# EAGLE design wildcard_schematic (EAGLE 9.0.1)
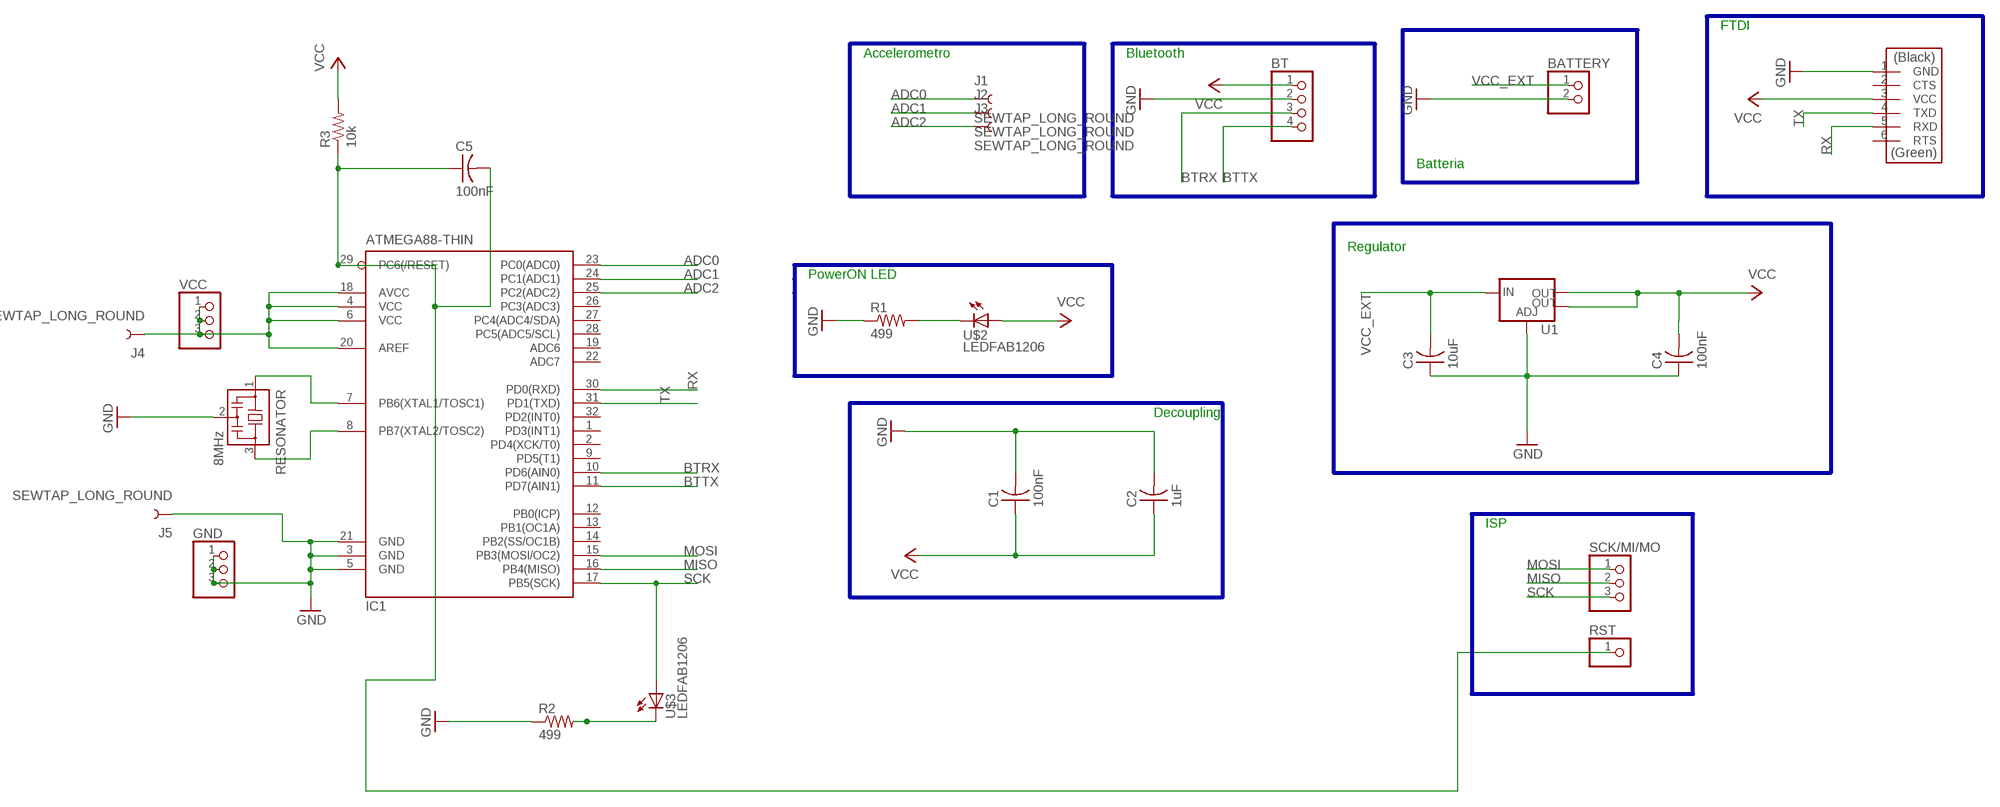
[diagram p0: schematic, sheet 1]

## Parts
BATTERY  PINHD-1X2  [1X02]
BT  PINHD-1X4  [1X04]
C1  100nF  CAP-US1206FAB  [C1206FAB]
C2  1uF  CAP-US1206FAB  [C1206FAB]
C3  10uF  CAP-US1206FAB  [C1206FAB]
C4  100nF  CAP-US1206FAB  [C1206FAB]
C5  100nF  CAP-US1206FAB  [C1206FAB]
GND  PINHD-1X3  [1X03]
IC1  ATMEGA88-THIN  [TQFP32-08THIN]
J1  SEWTAP_LONG_ROUND  [PETAL-LONG-2]
J2  SEWTAP_LONG_ROUND  [PETAL-LONG-2]
J3  SEWTAP_LONG_ROUND  [PETAL-LONG-2]
J4  SEWTAP_LONG_ROUND  [PETAL-LONG-2]
J5  SEWTAP_LONG_ROUND  [PETAL-LONG-2]
R1  499  RES-US1206FAB  [R1206FAB]
R2  499  RES-US1206FAB  [R1206FAB]
R3  10k  RES-US1206FAB  [R1206FAB]
RESONATOR  8MHz  RESONATOR  [EFOBM]
RST  PINHD-1X1  [1X01]
SCK/MI/MO  PINHD-1X3  [1X03]
U1  V_REG_LM1117SOT223  [SOT223]
U$2  LEDFAB1206  [LED1206FAB]
U$3  LEDFAB1206  [LED1206FAB]
U$4  FTDI-SMD-HEADER  [1X06SMD]
VCC  PINHD-1X3  [1X03]

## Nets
ADC0: IC1.23(PC0(ADC0)) J1.1
ADC1: IC1.24(PC1(ADC1)) J2.1
ADC2: IC1.25(PC2(ADC2)) J3.1
BTRX: BT.3 IC1.10(PD6(AIN0))
BTTX: BT.4 IC1.11(PD7(AIN1))
GND: BATTERY.2 BT.2 C1.2 C2.2 C3.1 C4.1 GND.1 GND.2 GND.3 IC1.3(GND) IC1.5(GND) IC1.21(GND) J5.1 R1.1 R2.1 RESONATOR.2 U1.1(ADJ) U$4.1(GND)
MISO: IC1.16(PB4(MISO)) SCK/MI/MO.2
MOSI: IC1.15(PB3(MOSI/OC2)) SCK/MI/MO.1
N$1: IC1.4(VCC) IC1.6(VCC) IC1.18(AVCC) IC1.20(AREF) J4.1 VCC.1 VCC.2 VCC.3
N$2: C5.1 C5.2 IC1.29(PC6(/RESET)) R3.1 RST.1
N$7: IC1.7(PB6(XTAL1/TOSC1)) RESONATOR.1
N$8: IC1.8(PB7(XTAL2/TOSC2)) RESONATOR.3
N$23: R2.2 U$3.2(C)
N$24: R1.2 U$2.2(C)
RX: IC1.30(PD0(RXD)) U$4.5(RXD)
SCK: IC1.17(PB5(SCK)) SCK/MI/MO.3 U$3.1(A)
TX: IC1.31(PD1(TXD)) U$4.4(TXD)
VCC: BT.1 C1.1 C2.1 C4.2 R3.2 U1.2(OUT) U1.4(OUT) U$2.1(A) U$4.3(VCC)
VCC_EXT: BATTERY.1 C3.2 U1.3(IN)
Unconnected: IC1.1(PD3(INT1)) IC1.2(PD4(XCK/T0)) IC1.9(PD5(T1)) IC1.12(PB0(ICP)) IC1.13(PB1(OC1A)) IC1.14(PB2(SS/OC1B)) IC1.19(ADC6) IC1.22(ADC7) IC1.26(PC3(ADC3)) IC1.27(PC4(ADC4/SDA)) IC1.28(PC5(ADC5/SCL)) IC1.32(PD2(INT0)) U$4.2(CTS) U$4.6(RTS)

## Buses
B$1
B$2
B$3
B$4
B$5
B$6
B$7
B$8

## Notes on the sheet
- FTDI
- Accelerometro | Bluetooth
- Batteria
- Regulator
- PowerON LED
- Decoupling
- ISP

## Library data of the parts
BATTERY = pinhead:PINHD-1X2: PIN HEADER
BT = pinhead:PINHD-1X4: PIN HEADER
C1-C5 = fab:CAP-US
GND SCK/MI/MO VCC = pinhead:PINHD-1X3: PIN HEADER
IC1 = fab:ATMEGA88-THIN
J1-J5 = LilyPad-Wearables:SEWTAP: SparkFun LilyPad Sew Taps
R1-R3 = fab:RES-US: Resistor (US Symbol)
RESONATOR = fab:RESONATOR
RST = pinhead:PINHD-1X1: PIN HEADER
U1 = fab:V_REG_LM1117: Voltage Regulator LM1117 Standard adjustable voltage regulator but in SMD form. Spark Fun Electronics SKU : COM-00595; PROD_ID: VREG-08170
U$2 U$3 = fab:LED: LED
U$4 = fab:FTDI-SMD-HEADER

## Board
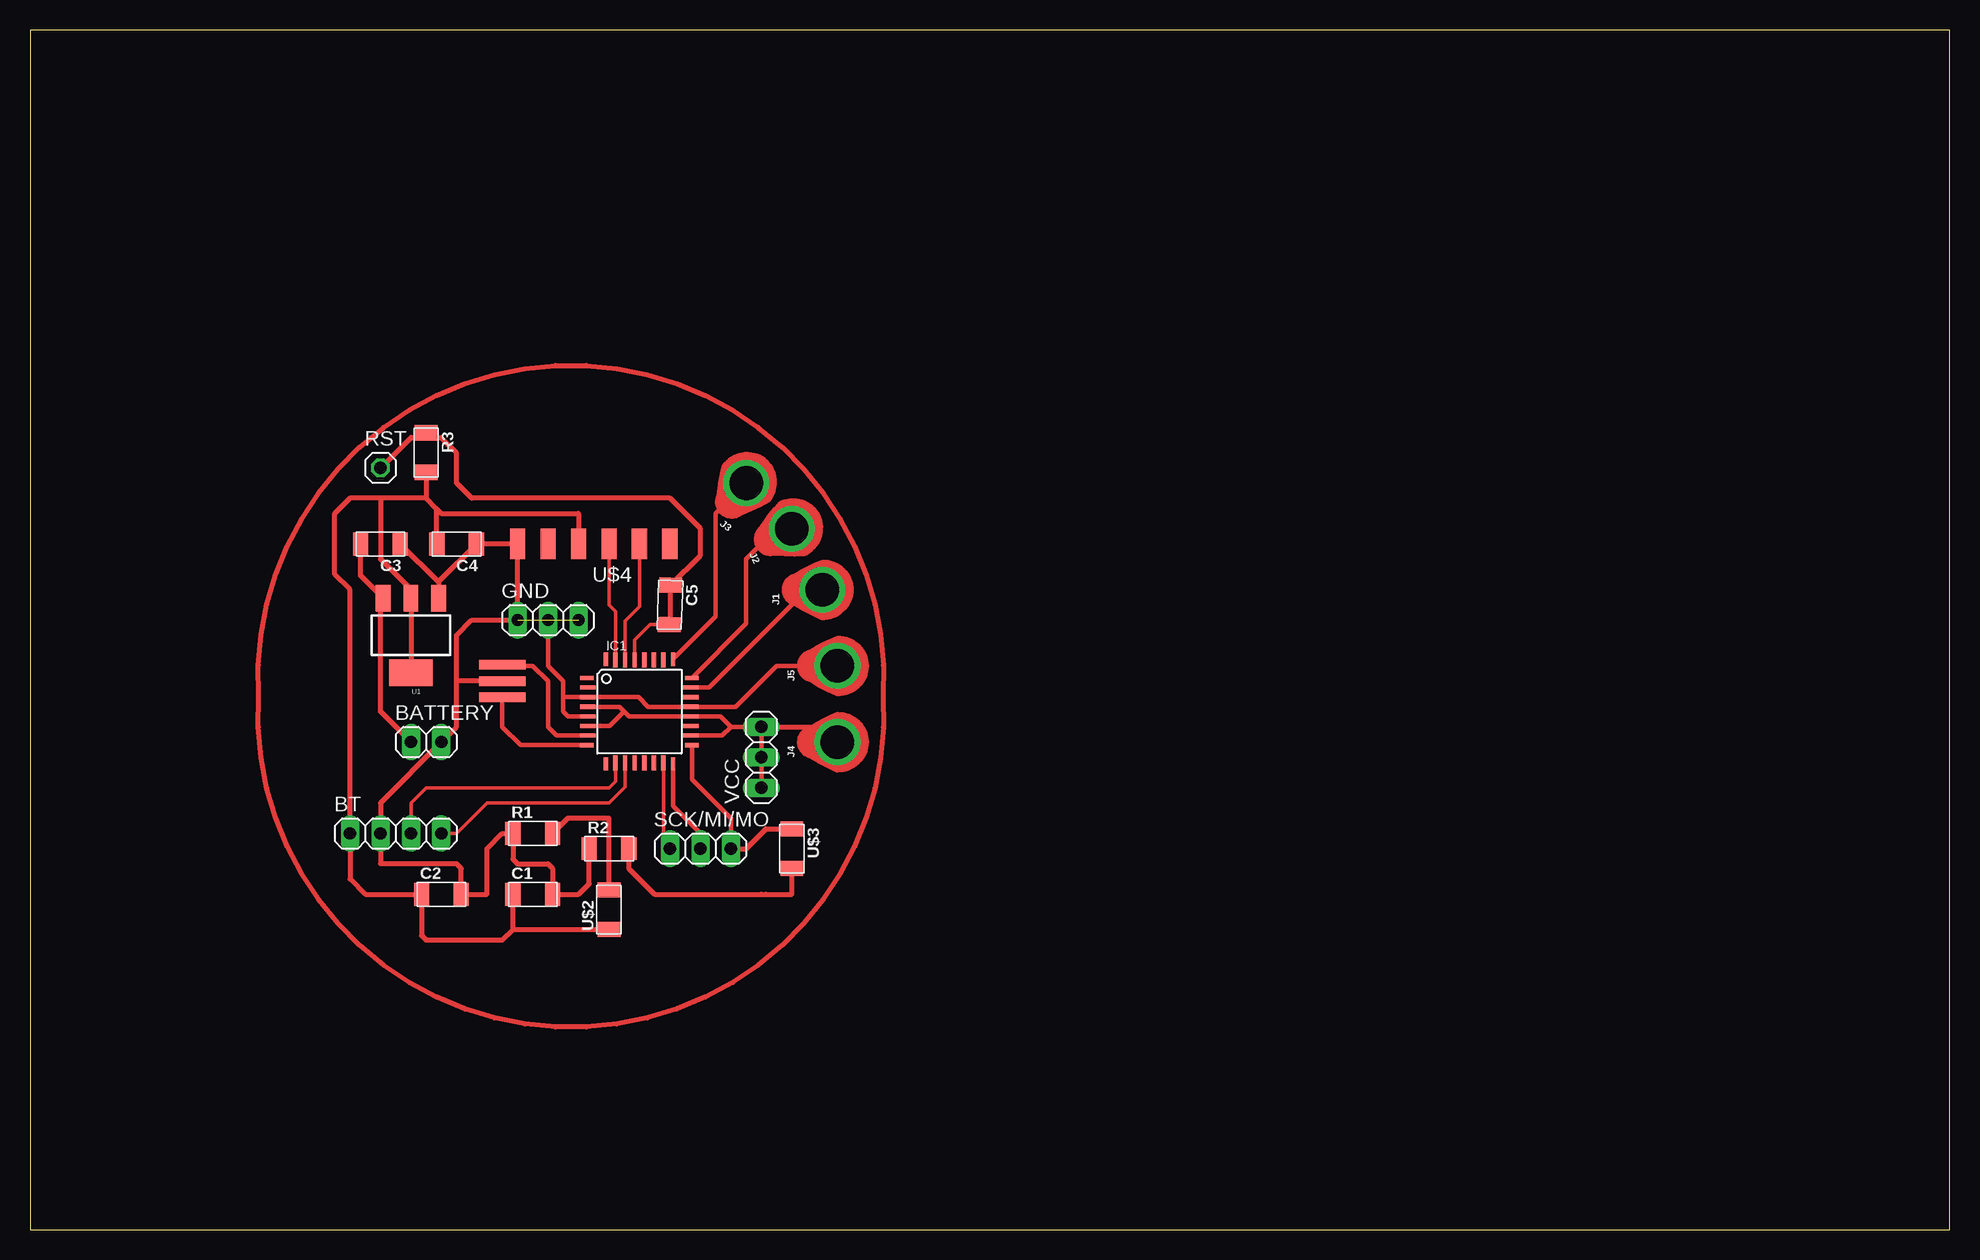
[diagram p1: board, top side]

Size 160 x 100 mm. Coordinates in mm from the lower left corner, seen from the top.
Outline: 0,0 160,0 160,100 0,100 0,0
Copper layers (1*16): Top 0.035mm / dielectric 1.5mm / Bottom 0.035mm
Design rules "default": minimum track width 6mil, minimum drill 0.35mm, track to track 6mil, track to pad 6mil, pad to pad 6mil, via to via 6mil, smd to smd 6mil, copper to edge 40mil, drill to drill 6mil, minimum pad ring 10mil, minimum via ring 8mil, stop-mask expansion 4mil, vias tented up to drill 0mil, thermal gap 10mil

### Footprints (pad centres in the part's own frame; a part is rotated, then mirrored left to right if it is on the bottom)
1X02 = drill 1.016 long: 1 -1.27,0; 2 1.27,0
1X04 = drill 1.016 long: 1 -3.81,0; 2 -1.27,0; 3 1.27,0; 4 3.81,0
C1206FAB = smd 1.27 x 1.905: 1 -1.651,0; 2 1.651,0
1X03 = drill 1.016 long: 1 -2.54,0; 2 0,0; 3 2.54,0
TQFP32-08THIN = smd 1.118 x 0.356: 1 -4.369,2.8; 8 -4.369,-2.8; 17 4.369,-2.8; 24 4.369,2.8 | smd 1.27 x 0.356: 2 -4.293,2; 3 -4.293,1.2; 4 -4.293,0.4; 5 -4.293,-0.4; 6 -4.293,-1.2; 7 -4.293,-2; 18 4.293,-2; 19 4.293,-1.2; 20 4.293,-0.4; 21 4.293,0.4; 22 4.293,1.2; 23 4.293,2 | smd 0.356 x 1.118: 9 -2.8,-4.369; 16 2.8,-4.369; 25 2.8,4.369; 32 -2.8,4.369 | smd 0.356 x 1.27: 10 -2,-4.293; 14 1.2,-4.293; 15 2,-4.293; 26 2,4.293; 27 1.2,4.293; 31 -2,4.293 | smd 0.35 x 1.27: 11 -1.2,-4.293; 12 -0.4,-4.293; 13 0.4,-4.293; 28 0.4,4.293; 29 -0.4,4.293; 30 -1.2,4.293
PETAL-LONG-2 = drill 2.794: 1 0,0
R1206FAB = smd 1.27 x 1.905: 1 -1.651,0; 2 1.651,0
EFOBM = smd 0.8 x 3.9: 1 -1.35,0; 2 0,0; 3 1.35,0
1X01 = drill 1.016 octagon: 1 0,0
SOT223 = smd 1.219 x 2.235: 1 -2.311,-3.099; 2 0,-3.099; 3 2.311,-3.099 | smd 3.6 x 2.2: 4 0,3.099
LED1206FAB = smd 1.27 x 1.905: 1 -1.651,0; 2 1.651,0
1X06SMD = smd 2.54 x 1.27: 1 0,6.35; 2 0,3.81; 3 0,1.27; 4 0,-1.27; 5 0,-3.81; 6 0,-6.35

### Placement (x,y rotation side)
BATTERY  33.02,40.64 0 top
BT  30.48,33.02 0 top
C1  41.91,27.94 0 top
C2  34.29,27.94 0 top
C3  29.21,57.15 180 top
C4  35.56,57.15 180 top
C5  53.34,52.07 268.1 top
GND  43.18,50.8 0 top
IC1  50.8,43.18 0 top
J1  66.04,53.34 90 top
J2  63.5,58.42 116.5 top
J3  59.69,62.23 143 top
J4  67.31,40.64 90 top
J5  67.31,46.99 90 top
J6  SEWTAP_LONG_ROUND  [PETAL-LONG-2]  not placed on the board
J7  SEWTAP_LONG_ROUND  [PETAL-LONG-2]  not placed on the board
R1  41.91,33.02 0 top
R2  48.26,31.75 0 top
R3  33.02,64.77 270 top
RESONATOR  39.37,45.72 270 top
RST  29.21,63.5 0 top
SCK/MI/MO  55.88,31.75 0 top
U1  31.75,49.53 180 top
U$2  48.26,26.67 90 top
U$3  63.5,31.75 270 top
U$4  46.99,57.15 90 top
VCC  60.96,39.37 90 top

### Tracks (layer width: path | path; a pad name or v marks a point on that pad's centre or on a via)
ADC0
  Top 0.356: IC1.23 56.61,45.18 64.77,53.34
  Top 0.406: 64.77,53.34 J1.1
ADC1
  Top 0.356: IC1.24 59.69,50.5 59.69,55.88 62.23,58.42
  Top 0.406: 62.23,58.42 J2.1
ADC2
  Top 0.356: IC1.25 57.15,51.1 57.15,59.69 58.42,60.96 59.69,60.96 J3.1
BTRX
  Top 0.305: BT.3 31.75,35.56 33.02,36.83 48.26,36.83 48.8,37.37 IC1.10
BTTX
  Top 0.305: BT.4 35.56,33.02 38.1,35.56 48.26,35.56 49.6,36.9 IC1.11
GND  (2 unrouted)
  Top 0.356: GND.2 43.18,46.99 44.45,45.72 44.45,44.45 | J5.1 62.23,46.99 58.82,43.58 IC1.21 52.07,43.58 51.67,43.58 51.53,43.58 50.73,44.38 IC1.3 44.52,44.38 44.45,44.45 | IC1.5 44.85,42.78 44.45,43.18 44.45,44.45
  Top 0.406: BT.2 29.21,35.56 BATTERY.2 35.56,41.91 35.56,45.72 | 29.21,31.75 BT.2 | 40.26,32.26 R1.1 | 46.61,30.99 R2.1 46.61,28.83 45.72,27.94 C1.2 43.56,30.1 43.18,30.48 40.64,30.48 40.26,30.86 R1.1 | 34.06,54 C4.1 U$4.1 GND.1 36.83,50.8 35.56,49.53 35.56,45.72 | 34.06,54 U1.1 | C3.1 34.01,54 34.06,54 | J5.1 66.04,46.99 | BT.2 29.21,30.48 35.56,30.48 35.94,30.1 C2.2 38.1,27.94 38.1,31.75 39.37,33.02 R1.1 | RESONATOR.2 35.56,45.72
MISO
  Top 0.356: IC1.16 53.6,35.3 55.88,33.02 SCK/MI/MO.2
MOSI
  Top 0.305: IC1.15 52.8,32.29 SCK/MI/MO.1
N$1
  Top 0.356: IC1.4 49.13,43.58 49.53,43.18 | 49.53,43.18 48.33,41.98 IC1.6 | 49.53,43.18 49.93,42.78 IC1.20 57.55,42.78 58.42,41.91 | 58.42,41.91 VCC.3 VCC.2 VCC.1 | IC1.18 57.69,41.18 58.42,41.91
  Top 0.406: VCC.3 66.04,41.91 J4.1
N$2
  Top 0.305: IC1.29 50.4,49.13 51.69,50.42 C5.2
  Top 0.406: R3.1 33.4,66.04 | 33.4,66.04 34.29,66.04 35.56,64.77 35.56,62.23 36.83,60.96 53.34,60.96 55.88,58.42 55.88,56.2 C5.1 53.4,50.53 C5.2 | RST.1 31.75,66.04 33.4,66.04
N$3
  Top 0.406: 19.05,44.45 arc-187 71.12,44.45 arc-187 19.05,44.45
N$7
  Top 0.356: RESONATOR.1 39.45,46.99 41.91,46.99 43.18,45.72 43.18,41.91 43.91,41.18 IC1.7
N$8
  Top 0.356: RESONATOR.3 39.37,41.91 40.9,40.38 IC1.8
N$23
  Top 0.406: 49.53,31.37 R2.2 49.91,30.1 52.07,27.94 60.96,27.94 61.34,27.94 63.5,27.94 U$3.2
N$24
  Top 0.406: U$2.2 48.26,34.29 44.83,34.29 R1.2
RX
  Top 0.305: IC1.30 49.6,50.73 50.8,51.93 U$4.5
SCK
  Top 0.356: IC1.17 55.17,37.54 58.42,34.29 SCK/MI/MO.3
  Top 0.406: 58.8,32.13 SCK/MI/MO.3 59.69,31.75 61.34,33.4 U$3.1
TX
  Top 0.305: U$4.4 48.26,52.07 48.8,51.53 IC1.31
VCC
  Top 0.406: U1.4 U1.2 31.75,53.34 29.21,55.88 29.21,60.96 | U$4.3 45.72,59.69 34.29,59.69 33.91,60.07 | C4.2 33.91,60.07 | 33.91,60.07 33.02,60.96 | 33.02,60.96 29.21,60.96 | 29.21,60.96 26.67,60.96 25.4,59.69 25.4,54.61 26.67,53.34 BT.1 26.67,29.21 27.94,27.94 C2.1 32.64,24.51 33.02,24.13 39.37,24.13 40.26,25.02 | R3.2 33.02,60.96 | 40.26,25.02 C1.1 | 40.26,25.02 U$2.1
VCC_EXT
  Top 0.406: BATTERY.1 29.21,43.18 29.21,52.4 U1.3 27.56,54.51 C3.2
